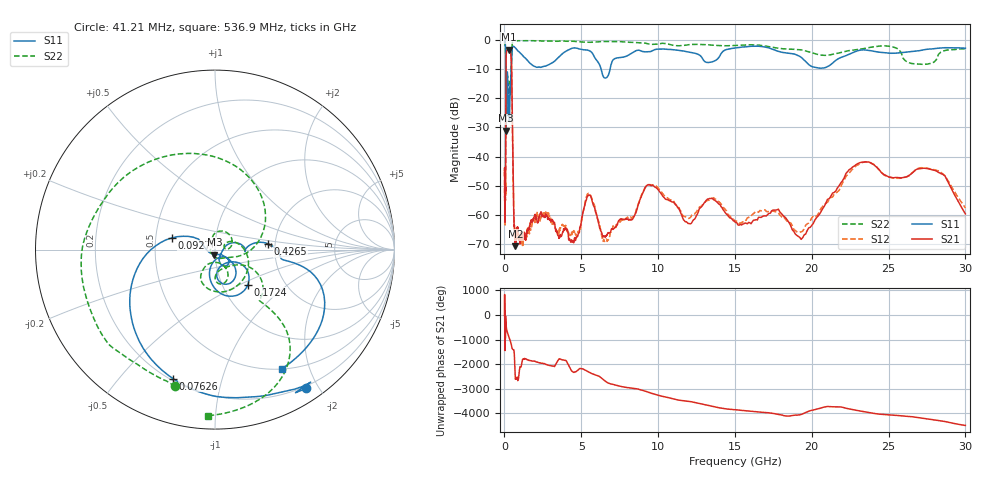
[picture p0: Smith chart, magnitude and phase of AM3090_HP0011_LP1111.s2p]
! Date/Time: Thu, Feb 28, 2019 1:57 PM
! Network Analyzer: Agilent Technologies E8364B Rev: A.07.50.67
! Sweep from 0.010 to 30.000 GHz, 1601 Points, Sweep Type: LOG
! Power Supply: 5.023 V, 0.002 A
# Hz S DB R 50
!freq MagS11 AngS11 MagS21 AngS21 MagS12 AngS12 MagS22 AngS22
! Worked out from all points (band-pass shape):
!   1601 points, 10 MHz to 30 GHz, reference 50 ohm
!   highest |S21| = -3.31 dB at 269.1 MHz (marker M1); lowest = -70.7 dB at 714.1 MHz (marker M2)
!   |S21| within 3 dB of the highest: 104.9 MHz to 441.5 MHz (336.6 MHz wide, 123 % of centre)
!   lowest |S11| = -31.1 dB at 100.9 MHz (marker M3), VSWR 1.06, Z = 49.6 - j2.74 ohm
!   |S11| at or under -10 dB: 91.56 MHz to 429.6 MHz (338 MHz wide, 130 % of centre); 6.289 GHz to 6.876 GHz (587.9 MHz wide, 8.93 % of centre)
!   |S22| runs from -31.9 to -0.2 dB; largest |S21 - S12| = 0.012
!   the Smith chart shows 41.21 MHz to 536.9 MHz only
!   S11 on the Smith chart (normalised r, x): 41.21 MHz: 0.17, -1.84; 76.26 MHz: 0.21, -0.70; 92.7 MHz: 0.61, +0.08; 172.4 MHz: 1.32, -0.55; 426.5 MHz: 1.84, +0.13; 536.9 MHz: 0.50, -1.59
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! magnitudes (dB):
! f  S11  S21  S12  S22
! 10 MHz  -0.2  -44.6  -46.6  -0.7
! 38.04 MHz  -0.5  -62.0  -60.2  -1.8
! 41.21 MHz  -0.7  -59.5  -62.4  -2.0
! 48.85 MHz  -0.8  -50.8  -48.5  -2.0
! 76.26 MHz  -2.4  -48.2  -47.1  -4.3
! 92.7 MHz  -12.0  -14.9  -14.9  -13.1
! 100.9 MHz  -31.1  -7.5  -7.5  -31.8
! 115.5 MHz  -14.1  -5.0  -4.9  -19.1
! 144.7 MHz  -19.5  -3.7  -3.6  -24.8
! 172.4 MHz  -11.5  -3.5  -3.5  -14.3
! 269.1 MHz  -20.4  -3.3  -3.3  -18.1
! 325.5 MHz  -27.9  -3.5  -3.5  -19.3
! 426.5 MHz  -10.5  -5.4  -5.4  -10.7
! 536.9 MHz  -2.4  -38.2  -38.0  -0.7
! 550.5 MHz  -2.3  -42.8  -42.7  -0.5
! 714.1 MHz  -2.8  -70.7  -69.4  -0.2
! 2.084 GHz  -9.4  -61.0  -60.9  -0.3
! 7.926 GHz  -5.6  -61.1  -61.0  -0.8
! 9.538 GHz  -4.0  -49.9  -49.6  -1.5
! 19.41 GHz  -6.4  -67.7  -65.5  -3.5
! 23.36 GHz  -3.4  -41.9  -41.9  -3.0
! 30 GHz  -2.9  -59.6  -57.6  -3.1
